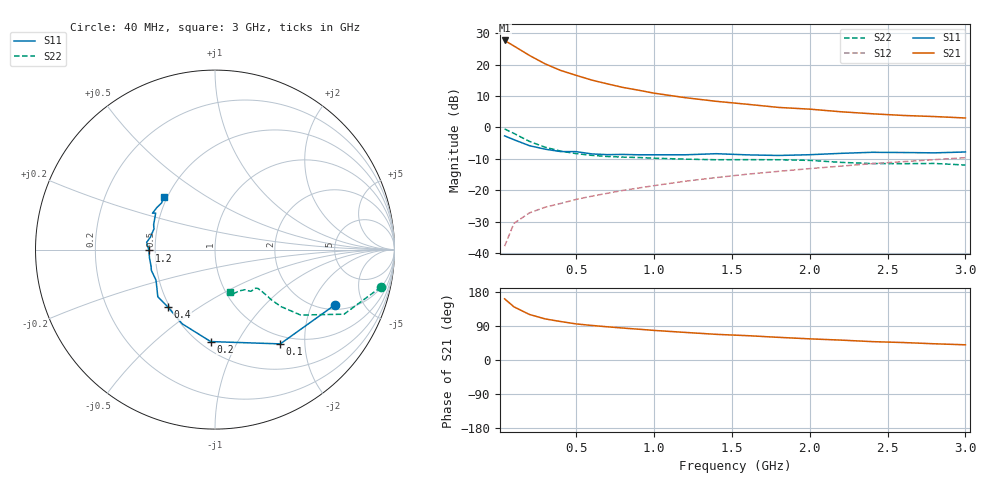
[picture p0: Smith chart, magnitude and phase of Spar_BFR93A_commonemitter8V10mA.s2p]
! Filename:  BFR93AF.S2P  Version:  2.0
! NXP part #: BFR93A  Date: May 1990
! Bias condition: Vce=8V, Ic=10mA
#  MHz  S  MA  R  50
! Freq  S11  S21  S12  S22  !GUM [dB]
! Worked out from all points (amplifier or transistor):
!   21 points, 40 MHz to 3 GHz, reference 50 ohm
!   highest |S21| = 27.7 dB at 40 MHz (marker M1)
!   |S21| within 3 dB of that: start of sweep to 141.1 MHz
!   unconditionally stable (mu >= 1): 931.9 MHz to 2.757 GHz
!   at 300 MHz: K = 0.66, MSG = 22.8 dB, |S12| = -25.4 dB
!   at 1 GHz: K = 1.02, MAG = 13.9 dB, |S12| = -18.5 dB
!   at 3 GHz: K = 0.99, MSG = 6.3 dB, |S12| = -9.6 dB
!   S11 on the Smith chart (normalised r, x): 40 MHz: 2.24, -3.01; 100 MHz: 0.87, -1.54; 200 MHz: 0.56, -0.78; 400 MHz: 0.49, -0.38; 1.2 GHz: 0.46, -0.00; 3 GHz: 0.48, +0.34
40  0.736 -24.7  24.13 161.4  0.013 77.8  0.948 -12.7
100  0.639 -55.3  19.7 140.2  0.03 65.6  0.804 -26.6
200  0.513 -92.7  13.93 120.1  0.044 58.4  0.6 -37.4
300  0.452 -113.9  10.26 108.5  0.054 57.0  0.486 -40.8
400  0.414 -129.2  8.059 101.5  0.062 58.5  0.421 -41.7
500  0.413 -140.5  6.731 95.2  0.072 60.1  0.384 -41.6
600  0.38 -149.0  5.659 91.2  0.081 61.7  0.361 -41.7
700  0.37 -152.9  4.933 87.6  0.09 64.4  0.346 -41.7
800  0.373 -161.9  4.329 84.3  0.1 65.1  0.338 -41.5
900  0.368 -165.5  3.911 81.3  0.109 66.5  0.333 -42.0
1000  0.368 -172.8  3.506 78.1  0.119 66.7  0.325 -42.0
1200  0.368 -179.3  2.975 72.8  0.14 67.7  0.314 -43.1
1400  0.383 173.9  2.603 67.7  0.16 67.7  0.307 -45.7
1600  0.367 169.3  2.335 64.2  0.181 68.5  0.308 -47.4
1800  0.359 161.2  2.083 59.8  0.201 67.7  0.307 -49.0
2000  0.369 157.9  1.955 55.8  0.222 67.5  0.3 -50.4
2200  0.388 148.4  1.777 52.5  0.243 67.9  0.279 -53.2
2400  0.403 149.8  1.651 48.5  0.266 66.3  0.267 -59.4
2600  0.4 144.1  1.552 46.1  0.286 65.5  0.266 -64.9
2800  0.395 138.9  1.491 42.8  0.308 64.4  0.268 -67.8
3000  0.408 134.4  1.415 40.1  0.331 63.2  0.253 -70.5
